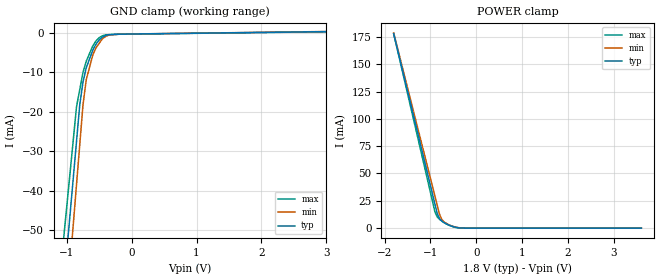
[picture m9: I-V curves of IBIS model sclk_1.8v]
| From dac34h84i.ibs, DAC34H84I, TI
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[Model] sclk_1.8v
Model_type Input
Vinl = 540.000mV
Vinh = 1.26000V
C_comp 641.000fF 640.000fF 642.000fF
| variable typ   min   max
[Voltage Range] 1.80000V 1.70000V 1.90000V
[POWER Clamp Reference] 1.80000V 1.70000V 1.90000V
[GND Clamp Reference] 0.00000V 0.00000V 0.00000V
[Temperature Range] 25   125   -40
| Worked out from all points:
|   GND clamp passes 1 mA (typ) near -0.43 V on its own axis
|   POWER clamp passes 1 mA (typ) near -0.47 V on its own axis
[GND Clamp]
-1.8V     -203.8mA   -230.4mA   -178.3mA
-850mV    -27.51mA   -38.44mA   -18.75mA
-800mV    -18.23mA   -28.34mA   -14.4mA
-750mV    -12.49mA   -18.24mA   -10.05mA
-700mV    -8.907mA   -11.91mA   -7.238mA
-600mV    -4.472mA   -5.718mA   -3.399mA
-550mV    -2.918mA   -3.837mA   -2.114mA
-500mV    -1.835mA   -2.698mA   -1.286mA
-450mV    -1.129mA   -1.559mA   -805.3uA
-350mV    -527.6uA   -634uA     -528.8uA
-175mV    -394.6uA   -386.1uA   -408.2uA
3.6V      366.4uA    395.9uA    323.2uA
[POWER Clamp]
-1.8V     177.9mA    178.6mA    177.9mA
-900mV    21.87mA    29.24mA    14.85mA
-850mV    13.2mA     20.95mA    10.28mA
-800mV    8.664mA    12.65mA    8.082mA
-750mV    6.386mA    7.907mA    6.582mA
-700mV    5.087mA    5.637mA    5.082mA
-600mV    2.916mA    3.083mA    2.768mA
-450mV    785.7uA    1.047mA    631.1uA
-300mV    105.5uA    97.64uA    57.61uA
3.6V      0A         0A         0A
